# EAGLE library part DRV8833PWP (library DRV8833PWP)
2A Low Voltage Dual Brushed DC or Single Bipolar Stepper Motor Driver (PWM Ctrl) Source: Datasheet
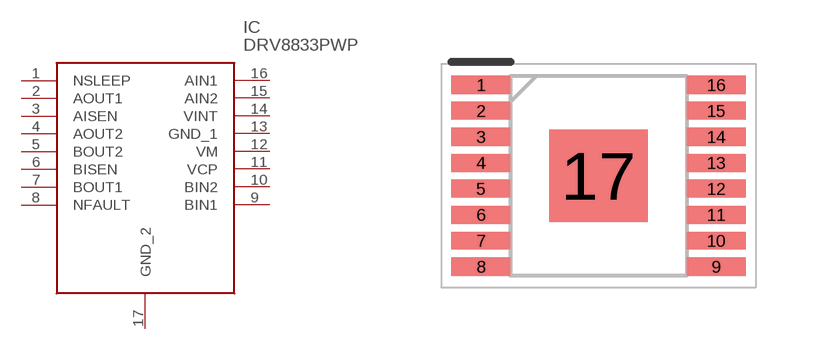
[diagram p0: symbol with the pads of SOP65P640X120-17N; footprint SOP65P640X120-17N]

Designator prefix IC

## DRV8833PWP (Description: 2A Low Voltage Dual Brushed DC or Single Bipolar Stepper Motor Driver (PWM Ctrl); Height: 1.2mm; Manufacturer_Name: Texas Instruments; Manufacturer_Part_Number: DRV8833PWP; Mouser_Part_Number: 595-DRV8833PWP; Mouser_Price-Stock: https://www.mouser.co.uk/ProductDetail/Texas-Instruments/DRV8833PWP?qs=luhu8ESwuKyOtvyRUEQSKQ%3D%3D)  [SOP65P640X120-17N]
1  NSLEEP
2  AOUT1
3  AISEN
4  AOUT2
5  BOUT2
6  BISEN
7  BOUT1
8  NFAULT
9  BIN1
10  BIN2
11  VCP
12  VM
13  GND_1
14  VINT
15  AIN2
16  AIN1
17  GND_2

## Footprint SOP65P640X120-17N (pad centres in mm)
PWP (R-PDSO-G16) (1)
smd 1.475 x 0.45: 1 -2.938,2.275; 2 -2.938,1.625; 3 -2.938,0.975; 4 -2.938,0.325; 5 -2.938,-0.325; 6 -2.938,-0.975; 7 -2.938,-1.625; 8 -2.938,-2.275; 9 2.938,-2.275; 10 2.938,-1.625; 11 2.938,-0.975; 12 2.938,-0.325; 13 2.938,0.325; 14 2.938,0.975; 15 2.938,1.625; 16 2.938,2.275
smd 2.46 x 2.31: 17 0,0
